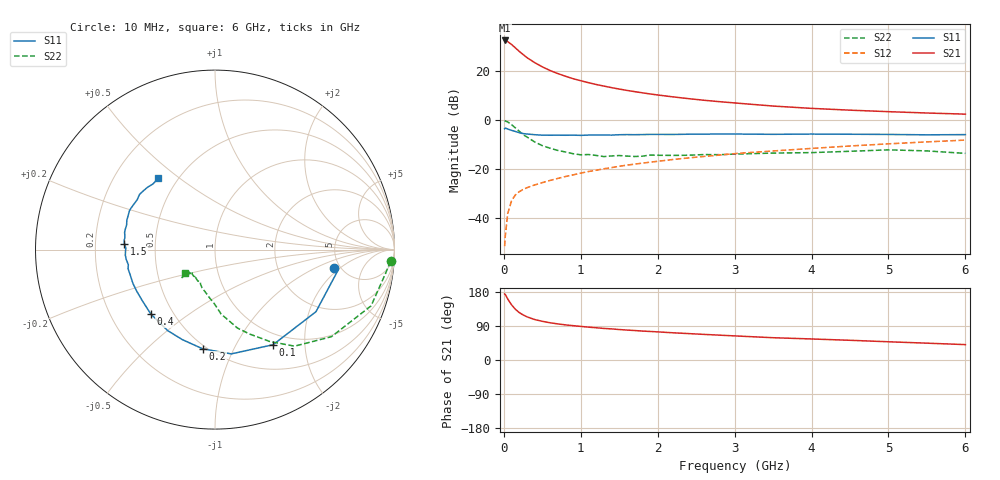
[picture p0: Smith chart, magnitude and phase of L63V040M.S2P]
!  INFINEON TECHNOLOGIES Small Signal Semiconductors
! BFR380L3 , Si-NPN RF-Transistor in TSLP-3-1
!  Vce=3 V,  Ic=40 mA
! Common Emitter S-Parameters:  07. March 2005
#  GHz  S  MA  R  50
! f  S11  S21  S12  S22
! GHz  Mag  Ang  Mag  Ang  Mag  Ang  Mag  Ang
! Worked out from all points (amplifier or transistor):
!   36 points, 10 MHz to 6 GHz, reference 50 ohm
!   highest |S21| = 32.5 dB at 10 MHz (marker M1)
!   |S21| within 3 dB of that: start of sweep to 149.3 MHz
!   unconditionally stable (mu >= 1): 1.629 GHz to 4.832 GHz
!   at 250 MHz: K = 0.47, MSG = 27.5 dB, |S12| = -28.2 dB
!   at 1.4 GHz: K = 0.99, MSG = 16.3 dB, |S12| = -19.3 dB
!   at 6 GHz: K = 0.98, MSG = 5.3 dB, |S12| = -8.1 dB
!   S11 on the Smith chart (normalised r, x): 10 MHz: 4.39, -1.65; 100 MHz: 0.83, -1.44; 200 MHz: 0.48, -0.76; 400 MHz: 0.38, -0.36; 1.5 GHz: 0.33, +0.03; 6 GHz: 0.39, +0.42
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0.01  0.6689 -8.9  42.24 174.3  0.0027 73.6  0.9801 -3.8
0.02  0.6922 -10.2  41.83 172.4  0.0045 87.2  0.9588 -8.1
0.05  0.6604 -31.6  39.96 161.1  0.0124 77.0  0.9245 -19.8
0.1  0.6209 -58.6  35 145.7  0.0227 67.6  0.8101 -36.8
0.15  0.5881 -81.1  29.84 133.8  0.03 59.7  0.6972 -50.5
0.2  0.5569 -97.1  25.33 125.2  0.0348 56.7  0.596 -59.2
0.25  0.5337 -109.8  21.82 119.0  0.0388 53.9  0.5084 -67.7
0.3  0.5228 -120.2  18.92 114.0  0.042 54.0  0.455 -74.0
0.4  0.5064 -135.1  14.93 106.8  0.0478 53.9  0.3605 -84.6
0.5  0.4949 -145.2  12.25 102.1  0.0533 55.5  0.3029 -90.5
0.6  0.4939 -152.5  10.31 98.3  0.059 56.7  0.2686 -96.8
0.7  0.4946 -157.9  8.947 95.3  0.0649 59.1  0.2419 -103.0
0.9  0.4959 -167.7  7.019 90.6  0.0767 61.6  0.2074 -113.1
1.1  0.4975 -173.6  5.813 86.7  0.0897 63.3  0.1995 -118.7
1.5  0.5054 176.4  4.313 80.4  0.1149 65.2  0.1903 -128.6
1.8  0.5091 170.7  3.617 76.4  0.1332 65.8  0.1844 -133.7
2.2  0.5112 164.4  2.987 71.8  0.1581 65.9  0.1914 -136.3
2.8  0.5234 155.7  2.388 65.6  0.1943 65.7  0.1981 -142.5
3.5  0.5149 147.3  1.942 58.8  0.2358 63.7  0.2135 -141.0
4.5  0.5169 141.2  1.601 52.0  0.2978 61.9  0.2322 -140.1
5.5  0.5031 133.3  1.401 44.4  0.3611 58.1  0.2365 -139.7
6  0.5082 128.3  1.328 40.6  0.393 56.0  0.2103 -141.9
